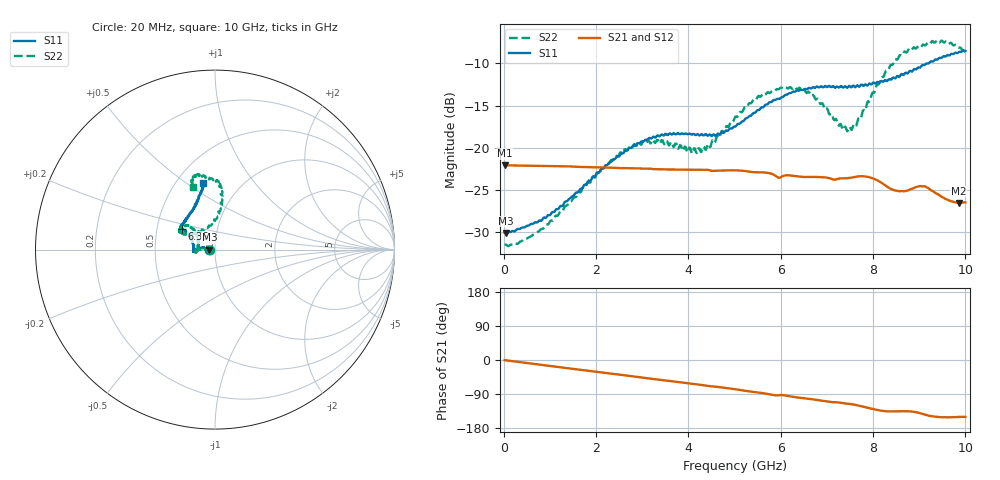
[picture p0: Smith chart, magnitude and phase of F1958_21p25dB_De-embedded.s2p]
! Integrated Device Technology
! Corporate Headquarters
! 6024 Silver Creek Valley Road
! San Jose, CA 95138  USA
! Phone:  1-408-284-8200
! Toll Free:  1-800-223-1366
! Webpage:  http://www.idt.com/
! Timing and RF Division
! 515 Groton Road, Suite 102
! Westford, MA 01886-6024
! Device:  F1958
! Description: 7-bit 0.25 dB Digital Step Attenuator
! Frequency:  0.001 -  6.000 GHz
! Package:  4x4 mm Thin QFN Plastic Package: 24 pin
! Ports:  2 RF, 12 DC
!  Pin  1  = D0
!  Pin  2  = VDD
!  Pin  3  = VMODE
!  Pin  4  = GND
!  Pin  5  = RF1  =  Port 1
!  Pin  6  = GND
!  Pin  7  = GND
!  Pin  8  = GND
!  Pin  9  = GND
!  Pin 10  = GND
!  Pin 11  = GND
!  Pin 12  = GND
!  Pin 13  = GND
!  Pin 14  = RF2  =  Port 2
!  Pin 15  = GND
!  Pin 16  = LE
!  Pin 17  = CLK
!  Pin 18  = DATA
!  Pin 19  = D6
!  Pin 20  = D5
!  Pin 21  = D4
!  Pin 22  = D3
!  Pin 23  = D2
!  Pin 24  = D1
! State:  85
! Atten State:  21.25 dB
! Voltage:  +3.30 Volts
! Current:  0.258 mA
! Data:  The device was measured on a F1958 evaluation board which has
!  individual transmission lines to the RF pins.  Data was collected
!  using a calibrated network analyzer.  The evaluation board was
!  de-embedded using Automatic Fixture Removal (AFR).
!  The reference plane is the edge of the package pin.
! Misc:
!  Action Tracker AT0419
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# GHz S dB R 50
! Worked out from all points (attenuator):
!   500 points, 20 MHz to 10 GHz, reference 50 ohm
!   highest |S21| = -22.06 dB at 20 MHz (marker M1); lowest = -26.5 dB at 9.86 GHz (marker M2)
!   lowest |S11| = -30.1 dB at 40 MHz (marker M3), VSWR 1.06, Z = 47 - j0.0413 ohm
!   |S11| at or under -10 dB: start of sweep to 9.159 GHz; 9.180494 GHz to 9.202776 GHz (22.28 MHz wide, 0.242 % of centre)
!   |S22| runs from -31.6 to -7.3 dB; largest |S21 - S12| = 0.00036
!   S11 on the Smith chart (normalised r, x): 20 MHz: 0.94, -0.00; 6.36 GHz: 0.67, +0.16; 10 GHz: 0.68, +0.58
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0.02  -30.03 -179.0  -22.06 -0.4  -22.06 -0.3  -31.47 -178.5
0.04  -30.07 -179.2  -22.06 -0.7  -22.06 -0.7  -31.44 -178.0
0.84  -28.46 170.8  -22.13 -13.2  -22.13 -13.2  -29.58 177.7
1.7  -24.80 170.8  -22.26 -26.3  -22.25 -26.3  -24.85 176.0
2.6  -20.57 176.7  -22.39 -40.0  -22.38 -40.1  -20.38 -179.2
3.36  -18.62 -175.8  -22.53 -51.9  -22.53 -52.0  -19.34 -171.6
4.24  -18.54 -179.3  -22.58 -65.1  -22.60 -65.2  -20.07 166.3
4.64  -18.30 171.6  -22.70 -71.0  -22.70 -71.0  -18.59 148.2
5.02  -17.47 160.6  -22.66 -77.3  -22.67 -77.3  -16.29 137.8
5.58  -15.22 150.4  -22.91 -86.8  -22.92 -86.8  -13.85 138.3
6.36  -13.21 147.9  -23.37 -98.9  -23.38 -98.8  -13.11 151.7
6.68  -12.88 146.5  -23.44 -103.5  -23.46 -103.4  -13.79 152.8
7.3  -12.69 140.8  -23.61 -113.0  -23.61 -112.9  -17.17 131.9
7.5  -12.71 138.2  -23.56 -116.1  -23.56 -116.0  -17.52 113.6
7.68  -12.68 135.3  -23.37 -119.9  -23.36 -119.9  -16.52 96.5
7.92  -12.38 129.1  -23.48 -127.1  -23.47 -127.1  -14.51 86.6
8.34  -11.88 119.1  -24.70 -135.8  -24.70 -135.9  -10.71 82.0
8.68  -11.25 112.4  -25.13 -135.2  -25.14 -135.1  -8.60 86.7
9.04  -10.39 107.0  -24.54 -140.9  -24.55 -141.1  -8.09 94.5
9.26  -9.75 104.8  -25.03 -148.1  -25.03 -148.2  -7.49 99.6
9.86  -8.67 99.9  -26.53 -150.2  -26.53 -150.1  -8.15 108.5
10  -8.53 99.9  -26.44 -150.2  -26.46 -150.2  -8.66 109.4
